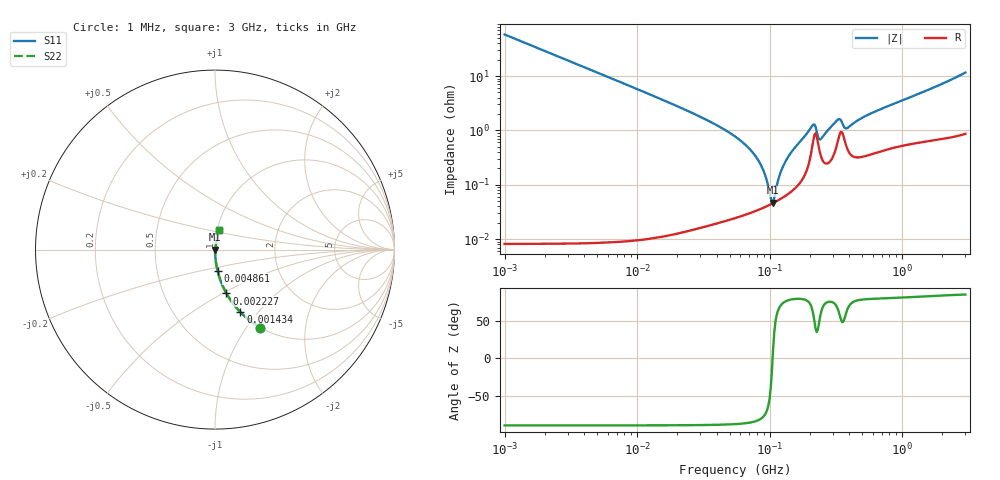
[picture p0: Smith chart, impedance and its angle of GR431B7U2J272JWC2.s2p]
!Murata Part Number: GR431B7U2J272JWC2
!These Parameters are Measured in Series Mode Connection
!Data Generated on Jun 10, 2025
!  o--ll--o
!Port1  Port2
!  o------o
!Operation Temp=25[degC], DC Bias Voltage=0[V]
!Freq. Start=1000[kHz] Stop=3[GHz] 401[Steps]
# Hz S RI R 50
!Freq.(Hz) S11(Real) S11(Imag) S21(Real) S21(Imag) S12(Real) S12(Imag) S22(Real) S22(Imag)
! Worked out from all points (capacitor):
!   401 points, 1 MHz to 3 GHz, reference 50 ohm
!   read as one part in series: C = 2.74 nF near 1.041 MHz
!   lowest |Z| = 46.7 mohm at 106 MHz (marker M1)
!   series resonance near 105.2 MHz, so ESL is about 840 pH
!   S11 on the Smith chart (normalised r, x): 1 MHz: 1.00, -1.16; 1.434 MHz: 1.00, -0.81; 2.227 MHz: 1.00, -0.52; 4.861 MHz: 1.00, -0.24; 3 GHz: 1.02, +0.23
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1000000  0.2527 -0.4345  0.7473 0.4345  0.7473 0.4345  0.2527 -0.4345
1433740  0.1413 -0.3482  0.8587 0.3482  0.8587 0.3482  0.1413 -0.3482
2226959  0.0639 -0.2443  0.9361 0.2443  0.9361 0.2443  0.0639 -0.2443
3823119  0.0226 -0.1485  0.9774 0.1485  0.9774 0.1485  0.0226 -0.1485
4861065  0.0141 -0.1177  0.9859 0.1177  0.9859 0.1177  0.0141 -0.1177
1.461624e7  0.00163 -0.0389  0.9984 0.0389  0.9984 0.0389  0.00163 -0.0389
5.477226e7  0.000303 -0.00775  0.9997 0.00775  0.9997 0.00775  0.000303 -0.00775
6.964249e7  0.000318 -0.00471  0.9997 0.00471  0.9997 0.00471  0.000318 -0.00471
8.173662e7  0.000351 -0.00285  0.9996 0.00285  0.9996 0.00285  0.000351 -0.00285
9.216659e7  0.000391 -0.00149  0.9996 0.00149  0.9996 0.00149  0.000391 -0.00149
1.018679e8  0.000437 -0.000367  0.9996 0.000367  0.9996 0.000367  0.000437 -0.000367
1.060286e8  0.000459 8.39e-05  0.9995 -8.39e-05  0.9995 -8.39e-05  0.000459 8.39e-05
1.195584e8  0.000542 0.00146  0.9995 -0.00146  0.9995 -0.00146  0.000542 0.00146
1.321429e8  0.000637 0.00265  0.9994 -0.00265  0.9994 -0.00265  0.000637 0.00265
2.094008e8  0.00504 0.011  0.995 -0.011  0.995 -0.011  0.00504 0.011
2.179536e8  0.00837 0.00959  0.9916 -0.00959  0.9916 -0.00959  0.00837 0.00959
2.361213e8  0.00462 0.00507  0.9954 -0.00507  0.9954 -0.00507  0.00462 0.00507
2.457655e8  0.00319 0.00633  0.9968 -0.00633  0.9968 -0.00633  0.00319 0.00633
3.252521e8  0.0062 0.0142  0.9938 -0.0142  0.9938 -0.0142  0.0062 0.0142
3.817355e8  0.00496 0.00968  0.995 -0.00968  0.995 -0.00968  0.00496 0.00968
8.005644e8  0.00533 0.028  0.9947 -0.028  0.9947 -0.028  0.00533 0.028
3e9  0.0214 0.112  0.9786 -0.112  0.9786 -0.112  0.0214 0.112
